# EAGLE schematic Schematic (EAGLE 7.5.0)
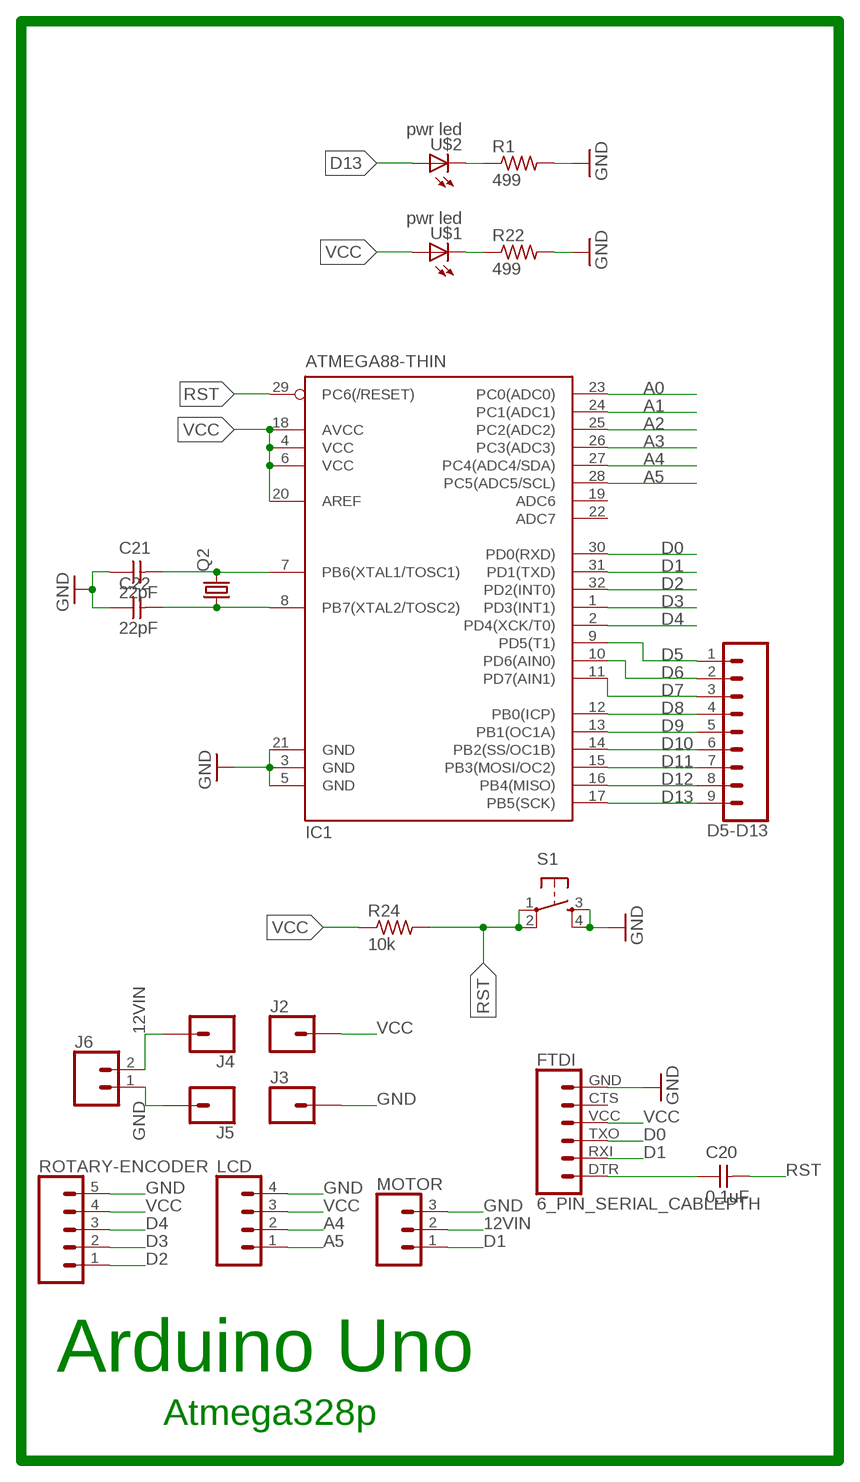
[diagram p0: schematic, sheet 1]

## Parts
C20  0.1uF  CAP-UNPOLARIZEDFAB  [C1206FAB]
C21  22pF  CAP-UNPOLARIZEDFAB  [C1206FAB]
C22  22pF  CAP-UNPOLARIZEDFAB  [C1206FAB]
D5-D13  CONN_09  [1X09]
FTDI  6_PIN_SERIAL_CABLEPTH  [FTDI_BASIC]
IC1  ATMEGA88-THIN  [TQFP32-08THIN]
J2  CONN_01  [1X01]
J3  CONN_01  [1X01]
J4  CONN_01  [1X01]
J5  CONN_01  [1X01]
J6  CONN_02PTH4  [1X02_XTRA_BIG]
LCD  CONN_04  [1X04]
MOTOR  CONN_03  [1X03]
Q2  CRYSTALHC49U-V  [HC49U-V]
R1  499  RES-US1206FAB  [R1206FAB]
R22  499  RES-US1206FAB  [R1206FAB]
R24  10k  RES-US1206FAB  [R1206FAB]
ROTARY-ENCODER  CONN_05  [1X05]
S1  6MM_SWITCH6MM_SWITCH  [6MM_SWITCH]
U$1  pwr led  LEDFAB1206  [LED1206FAB]
U$2  pwr led  LEDFAB1206  [LED1206FAB]

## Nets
12VIN: J4.1 J6.2 MOTOR.2
A0: IC1.23(PC0(ADC0))
A1: IC1.24(PC1(ADC1))
A2: IC1.25(PC2(ADC2))
A3: IC1.26(PC3(ADC3))
A4: IC1.27(PC4(ADC4/SDA)) LCD.2
A5: IC1.28(PC5(ADC5/SCL)) LCD.1
D0: FTDI.TXO IC1.30(PD0(RXD))
D1: FTDI.RXI IC1.31(PD1(TXD)) MOTOR.1
D2: IC1.32(PD2(INT0)) ROTARY-ENCODER.1
D3: IC1.1(PD3(INT1)) ROTARY-ENCODER.2
D4: IC1.2(PD4(XCK/T0)) ROTARY-ENCODER.3
D5: D5-D13.1 IC1.9(PD5(T1))
D6: D5-D13.2 IC1.10(PD6(AIN0))
D7: D5-D13.3 IC1.11(PD7(AIN1))
D8: D5-D13.4 IC1.12(PB0(ICP))
D9: D5-D13.5 IC1.13(PB1(OC1A))
D10: D5-D13.6 IC1.14(PB2(SS/OC1B))
D11: D5-D13.7 IC1.15(PB3(MOSI/OC2))
D12: D5-D13.8 IC1.16(PB4(MISO))
D13: D5-D13.9 IC1.17(PB5(SCK)) U$2.1(A)
GND: C21.1 C22.1 FTDI.GND IC1.3(GND) IC1.5(GND) IC1.21(GND) J3.1 J5.1 J6.1 LCD.4 MOTOR.3 R1.2 R22.2 ROTARY-ENCODER.5 S1.3(S) S1.4(S1)
N$1: R1.1 U$2.2(C)
N$10: C21.2 IC1.7(PB6(XTAL1/TOSC1)) Q2.2
N$11: C22.2 IC1.8(PB7(XTAL2/TOSC2)) Q2.1
N$12: R22.1 U$1.2(C)
N$17: C20.1 FTDI.DTR
RST: C20.2 IC1.29(PC6(/RESET)) R24.2 S1.1(P) S1.2(P1)
VCC: FTDI.VCC IC1.4(VCC) IC1.6(VCC) IC1.18(AVCC) IC1.20(AREF) J2.1 LCD.3 R24.1 ROTARY-ENCODER.4 U$1.1(A)
Unconnected: FTDI.CTS IC1.19(ADC6) IC1.22(ADC7)

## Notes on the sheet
- Arduino Uno
- Atmega328p

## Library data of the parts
C20-C22 = fab:CAP-UNPOLARIZED
D5-D13 = SparkFun-Connectors:CONN_09: Multi connection point. Often used as Generic Header-pin footprint for 0.1 inch spaced/style header connections On any of the 0.1 inch spaced packages, you can populate with these: Break Away Headers - Straight (PRT-00116) Break Away Male Headers - Right Angle (PRT-00553) Female Headers (PRT-00115)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
FTDI = SparkFun-Connectors:6_PIN_SERIAL_CABLE: 6-pin header connection for use with the "FTDI BASIC" pinout - CABLE SIDE. Also known as "Arduino Serial Program Header". This is used on a design to provide a 6-pin connection point for serial communication usually from a USB cable (D+/D-) to these headers (RX/TX). It also has the remaining pins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
IC1 = fab:ATMEGA88-THIN
J2-J5 = SparkFun-Connectors:CONN_01: Single connection point. Often used as Generic Header-pin footprint for 0.1 inch spaced/style header connections
J6 = SparkFun-Connectors:CONN_02: Multi connection point. Often used as Generic Header-pin footprint for 0.1 inch spaced/style header connections
LCD = SparkFun-Connectors:CONN_04: Multi connection point. Often used as Generic Header-pin footprint for 0.1 inch spaced/style header connections On any of the 0.1 inch spaced packages, you can populate with these: Break Away Headers - Straight (PRT-00116) Break Away Male Headers - Right Angle (PRT-00553) Female Headers (PRT-00115)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; PROD_ID: CONN-09696
MOTOR = SparkFun-Connectors:CONN_03: Multi connection point. Often used as Generic Header-pin footprint for 0.1 inch spaced/style header connections On any of the 0.1 inch spaced packages, you can populate with these: Break Away Headers - Straight (PRT-00116) Break Away Male Headers - Right Angle (PRT-00553) Female Headers (PRT-00115)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; PROD_ID: XXX-00000; VALUE: 455-1750-1-ND
Q2 = adafruit:CRYSTAL: CRYSTAL; OC_FARNELL: 1666969; OC_NEWARK: unknown
R1 R22 R24 = fab:RES-US: Resistor (US Symbol)
ROTARY-ENCODER = SparkFun-Connectors:CONN_05: Multi connection point. Often used as Generic Header-pin footprint for 0.1 inch spaced/style header connections On any of the 0.1 inch spaced packages, you can populate with these: Break Away Headers - Straight (PRT-00116) Break Away Male Headers - Right Angle (PRT-00553) Female Headers (PRT-00115)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
S1 = fab:6MM_SWITCH: OMRON SWITCH
U$1 U$2 = fab:LED: LED

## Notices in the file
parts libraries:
SparkFun-Connectors: Licensing: Creative Commons ShareAlike 4.0 International - https://creativecommons.org/licenses/by-sa/4.0
